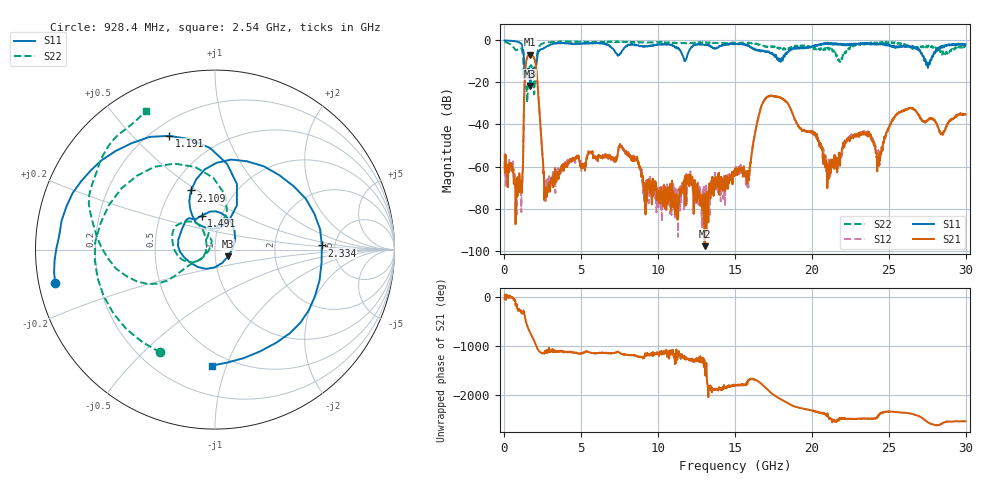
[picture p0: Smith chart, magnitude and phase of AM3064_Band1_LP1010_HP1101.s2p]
# Hz S DB R 50.0
!freq dBS11 angS11 dBS21 angS21 dBS12 angS12 dBS22 angS22
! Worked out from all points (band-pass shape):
!   1600 points, 10 MHz to 29.98 GHz, reference 50 ohm
!   highest |S21| = -6.72 dB at 1.678 GHz (marker M1); lowest = -97.9 dB at 13.02 GHz (marker M2)
!   |S21| within 3 dB of the highest: 1.42 GHz to 1.986 GHz (565.9 MHz wide, 33.2 % of centre)
!   lowest |S11| = -21.7 dB at 1.678 GHz (marker M3), VSWR 1.18, Z = 57.7 - j4.29 ohm
!   |S11| at or under -10 dB: 1.277 GHz to 2.095 GHz (818 MHz wide, 48.5 % of centre); 17.95742 GHz to 17.98708 GHz (29.67 MHz wide, 0.165 % of centre); 27.4 GHz to 27.68 GHz (281.2 MHz wide, 1.02 % of centre)
!   |S22| runs from -29.6 to -0.4 dB; largest |S21 - S12| = 0.0074
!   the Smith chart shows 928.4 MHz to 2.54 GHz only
!   S11 on the Smith chart (normalised r, x): 928.4 MHz: 0.05, -0.10; 1.191 GHz: 0.27, +0.64; 1.491 GHz: 0.81, +0.32; 2.109 GHz: 0.63, +0.47; 2.334 GHz: 3.92, +0.28; 2.54 GHz: 0.40, -0.89
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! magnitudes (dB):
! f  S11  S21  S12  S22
! 10 MHz  0.0  -58.0  -53.8  -0.4
! 928.4 MHz  -0.8  -65.2  -64.9  -3.8
! 1.191 GHz  -3.3  -62.1  -60.9  -6.5
! 1.491 GHz  -13.9  -7.9  -7.9  -28.9
! 1.678 GHz  -21.7  -6.7  -6.7  -12.2
! 2.109 GHz  -9.0  -16.7  -16.6  -7.6
! 2.334 GHz  -4.5  -39.9  -40.0  -2.2
! 2.54 GHz  -3.8  -63.4  -63.4  -1.3
! 5.015 GHz  -1.5  -61.1  -61.5  -0.7
! 7.582 GHz  -6.0  -50.3  -50.6  -0.7
! 10 GHz  -2.0  -73.5  -70.0  -1.0
! 11.97 GHz  -5.7  -63.9  -67.1  -1.3
! 13.02 GHz  -2.3  -97.9  -75.8  -1.1
! 15 GHz  -1.7  -60.8  -62.8  -1.4
! 15.85 GHz  -2.5  -65.8  -66.7  -1.3
! 17.14 GHz  -5.6  -26.7  -26.8  -3.2
! 19.99 GHz  -3.2  -43.5  -43.3  -3.1
! 21.08 GHz  -1.9  -59.3  -56.6  -4.2
! 23.18 GHz  -1.2  -44.2  -44.2  -2.0
! 24.36 GHz  -1.8  -55.7  -57.6  -1.5
! 25 GHz  -2.0  -42.0  -42.1  -1.0
! 29.98 GHz  -1.8  -35.2  -34.8  -3.2
